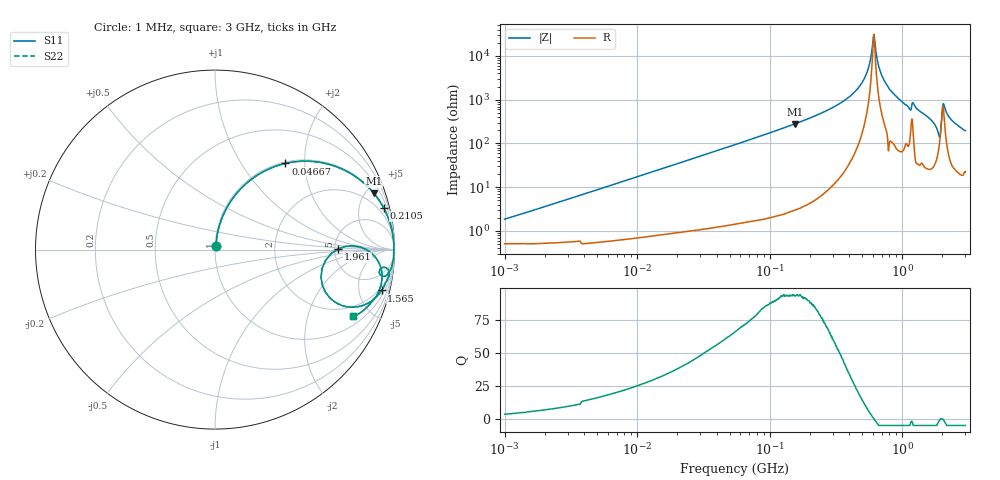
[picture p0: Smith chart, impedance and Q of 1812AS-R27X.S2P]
!s-Parameter Generated by FASTRON Sdn. Bhd.
!FASTRON P/N : 1812AS-R27X
!Keysight Technologies,E4991B,MY54100416,A.01.15
!Date created: Fri Oct 13 15:05:03 2023
!Version  : Rev00 Fri Oct 13 15:05:03 2023
!Data & Calibration Information:
!Freq	S11	S21	S12	S22
!PortZ  Port1:50+j0  Port2:50+j0
!When reading, reference impedance value at option line is always used.
! Remarks : This data is being provided solely for informational purposes.
# Hz S dB R 50
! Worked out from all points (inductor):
!   1601 points, 1 MHz to 3 GHz, reference 50 ohm
!   read as one part in series: L = 284 nH near 1.041 MHz
!   highest Q = 93.6 at 155.1 MHz (marker M1), where L = 288 nH
!   self-resonance near 611 MHz
!   S11 on the Smith chart (normalised r, x): 1 MHz: 1.01, +0.04; 46.67 MHz: 1.03, +1.60; 210.5 MHz: 1.09, +8.07; 1.565 GHz: 1.52, -7.99; 1.961 GHz: 5.39, +0.09; 3 GHz: 1.45, -3.91
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1000000  -34.64 73.0  -0.05 -1.0  -0.05 -1.0  -34.64 73.0
3804036  -23.54 81.8  -0.06 -3.8  -0.06 -3.8  -23.54 81.8
1.447069e7  -12.39 74.3  -0.33 -13.9  -0.33 -13.9  -12.39 74.3
4.666789e7  -4.16 50.8  -2.22 -38.3  -2.22 -38.3  -4.16 50.8
5.477226e7  -3.35 46.3  -2.82 -42.8  -2.82 -42.8  -3.35 46.3
1.550909e8  -0.55 19.5  -9.51 -69.8  -9.51 -69.8  -0.55 19.5
2.083556e8  -0.29 14.0  -12.30 -75.3  -12.30 -75.3  -0.29 14.0
2.104513e8  -0.28 13.9  -12.40 -75.5  -12.40 -75.5  -0.28 13.9
3.402349e8  -0.08 6.9  -18.46 -82.0  -18.46 -82.0  -0.08 6.9
4.593788e8  -0.04 3.2  -24.95 -84.0  -24.95 -84.0  -0.04 3.2
5.418594e8  -0.03 1.4  -32.42 -81.6  -32.42 -81.6  -0.03 1.4
6.110031e8  -0.03 0.0  -49.85 -2.7  -49.85 -2.7  -0.03 0.0
6.855309e8  -0.03 -1.3  -32.74 79.8  -32.74 79.8  -0.03 -1.3
7.925923e8  -0.03 -3.1  -25.34 84.5  -25.34 84.5  -0.03 -3.1
1.11944e9  -0.26 -8.3  -16.74 74.2  -16.74 74.2  -0.26 -8.3
1.231095e9  -0.19 -7.3  -17.90 76.6  -17.90 76.6  -0.19 -7.3
1.565327e9  -0.39 -13.8  -12.44 72.5  -12.44 72.5  -0.39 -13.8
1.86495e9  -2.22 -23.8  -7.40 47.0  -7.40 47.0  -2.22 -23.8
1.960646e9  -3.26 0.4  -10.08 -0.8  -10.08 -0.8  -3.26 0.4
2.081985e9  -0.61 -6.6  -17.70 55.2  -17.70 55.2  -0.61 -6.6
2.359433e9  -0.57 -15.7  -11.30 68.8  -11.30 68.8  -0.57 -15.7
3e9  -1.38 -25.5  -7.26 58.0  -7.26 58.0  -1.38 -25.5
